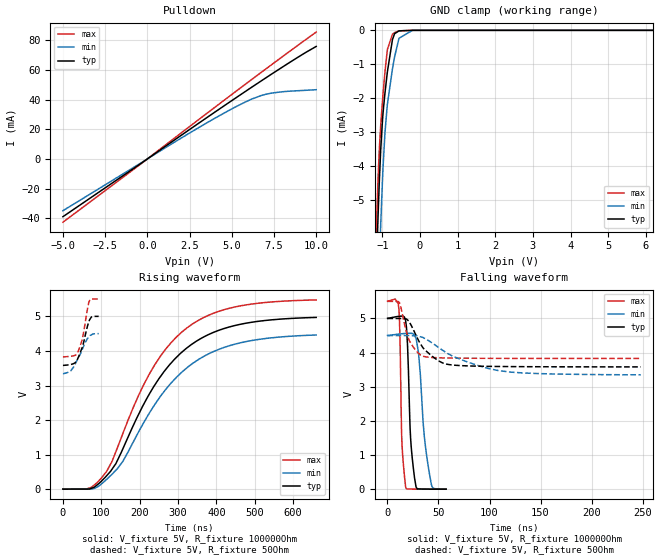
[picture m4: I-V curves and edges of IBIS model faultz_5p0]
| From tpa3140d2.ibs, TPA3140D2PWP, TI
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|   faultz_5p0 Model
[Model]   faultz_5p0
Model_type   Open_drain
Polarity   Non-Inverting
Vmeas = 2.5
Vref = 5
Cref = 2pF
Rref = 100000
|   typ   min   max
|   (nom PVT)   (fast PVT)   (slow PVT)
C_comp   1.652e-13   1.528e-13   1.897e-13
| Where nom  PVT is Nominal Process, 5V, 27C
|   Fast PVT is Strong Process,  5.5V, -40C
|   Slow PVT is Weak Process,   4.5V, 125C
[Voltage Range]   5   4.5   5.5
|Junction Temperature
[Temperature Range]   27   125   -40
[Pullup Reference]   5   4.5   5.5
[Pulldown Reference]   0   0   0
[Power Clamp Reference]   5   4.5   5.5
[GND Clamp Reference]   0   0   0
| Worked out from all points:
|   slope of the pulldown table from 0 to 0.75 V, typ, clamps not added: 125 ohm
|   GND clamp passes 1 mA (typ) near -0.83 V on its own axis
|   falling waveform, V_fixture 5V, R_fixture 100000Ohm: 20-80 % time 4.08ns typ, 7.25ns min, 2.41ns max; typ from 5 V to 0.008 V
|   rising waveform, V_fixture 5V, R_fixture 100000Ohm: 20-80 % time 162ns typ, 169ns min, 156ns max; typ from 0.006 V to 4.97 V
|   falling waveform, V_fixture 5V, R_fixture 50Ohm: 20-80 % time 20.4ns typ, 49.2ns min, 11ns max; typ from 5 V to 3.58 V
|   rising waveform, V_fixture 5V, R_fixture 50Ohm: 20-80 % time 21.9ns typ, 29.6ns min, 17.6ns max; typ from 3.58 V to 5 V
[Pulldown]
|   Voltage   I(typ)   I(min)   I(max)
-5V       -38.96mA   -34.91mA   -42.67mA
-486mV    -3.844mA   -3.412mA   -4.216mA
2.421V    19.27mA    16.98mA    21.21mA
4.284V    33.86mA    29.33mA    37.36mA
5.72V     44.93mA    37.99mA    49.71mA
6.75V     52.75mA    42.86mA    58.5mA
7.312V    56.97mA    44.37mA    63.27mA
8.223V    63.68mA    45.6mA     70.94mA
10V       75.98mA    46.75mA    85.67mA
[GND Clamp]
|   Voltage   I(typ)   I(min)   I(max)
-5V       -185mA     -178.6mA   -197.8mA
-1.21V    -8.9mA     -11.54mA   -7.747mA
-1.149V   -6.665mA   -9.293mA   -5.497mA
-1.115V   -5.498mA   -8.066mA   -4.397mA
-1.045V   -3.544mA   -5.766mA   -2.815mA
-980mV    -2.414mA   -3.999mA   -1.851mA
-931.5mV  -1.854mA   -3.027mA   -1.237mA
-874.5mV  -1.3mA     -2.269mA   -644.9uA
-731.5mV  -274uA     -1.132mA   -114.2uA
-558mV    -15.73uA   -233.2uA   -15.08uA
-200mV    -11.26nA   -128.7nA   0A
10V       0A         0A         0A
[POWER Clamp]
|   Voltage   I(typ)   I(min)   I(max)
-5V       0A         0A         0A
0V        0A         0A         0A
10V       0A         0A         0A
[Ramp]
R_load = 100000
|   typ   min   max
dV/dt_r   2.98395/1.62882e-07   2.68046/1.70264e-07   3.28666/1.56129e-07
dV/dt_f   2.99623/4.08354e-09   2.69603/7.2672e-09   3.29623/2.41461e-09
[Falling Waveform]
V_fixture = 5V
V_fixture_min = 4.5V
V_fixture_max = 5.5V
R_fixture = 100000Ohm
|   Time   V(typ)   V(min)   V(max)
0s        5V         4.5V       5.5V
11.25ns   5.064V     4.543V     5.264V
14ns      5.069V     4.553V     1.487V
17.94ns   4.894V     4.563V     56.07mV
19.65ns   4.223V     4.568V     14.83mV
22.7ns    1.48V      4.566V     11.08mV
27.99ns   71.73mV    4.417V     9.307mV
36.04ns   10.42mV    1.571V     8.281mV
42.81ns   8.808mV    174.7mV    8.092mV
57.48ns   7.746mV    10.93mV    7.54mV
[Rising Waveform]
V_fixture = 5V
V_fixture_min = 4.5V
V_fixture_max = 5.5V
R_fixture = 100000Ohm
|   Time   V(typ)   V(min)   V(max)
0s        6.249mV    6.297mV    6.259mV
74.83ns   30.07mV    10.25mV    60.01mV
114ns     393.1mV    286.8mV    519.4mV
156ns     1.166V     804.8mV    1.608V
226ns     2.769V     2.219V     3.349V
268ns     3.465V     2.89V      4.056V
324ns     4.095V     3.521V     4.673V
375.9ns   4.456V     3.894V     5.013V
450ns     4.74V      4.202V     5.276V
660ns     4.969V     4.461V     5.476V
[Falling Waveform]
V_fixture = 5V
V_fixture_min = 4.5V
V_fixture_max = 5.5V
R_fixture = 50Ohm
|   Time   V(typ)   V(min)   V(max)
0s        5V         4.5V       5.5V
11.88ns   5V         4.5V       5.455V
18.64ns   4.984V     4.5V       4.597V
21.34ns   4.901V     4.5V       4.352V
29.82ns   4.395V     4.484V     3.997V
36.04ns   4.104V     4.423V     3.885V
50.01ns   3.761V     4.153V     3.851V
57.93ns   3.664V     3.993V     3.845V
108.8ns   3.596V     3.476V     3.833V
248.2ns   3.584V     3.351V     3.83V
[Rising Waveform]
V_fixture = 5V
V_fixture_min = 4.5V
V_fixture_max = 5.5V
R_fixture = 50Ohm
|   Time   V(typ)   V(min)   V(max)
0s        3.583V     3.342V     3.83V
20.87ns   3.61V      3.431V     3.846V
31.12ns   3.653V     3.603V     3.871V
36.04ns   3.722V     3.71V      3.91V
49.26ns   4.073V     4.014V     4.29V
54.4ns    4.267V     4.15V      4.561V
64.57ns   4.743V     4.366V     5.262V
67.64ns   4.848V     4.407V     5.417V
74.16ns   4.982V     4.467V     5.498V
93.08ns   5V         4.5V       5.5V
